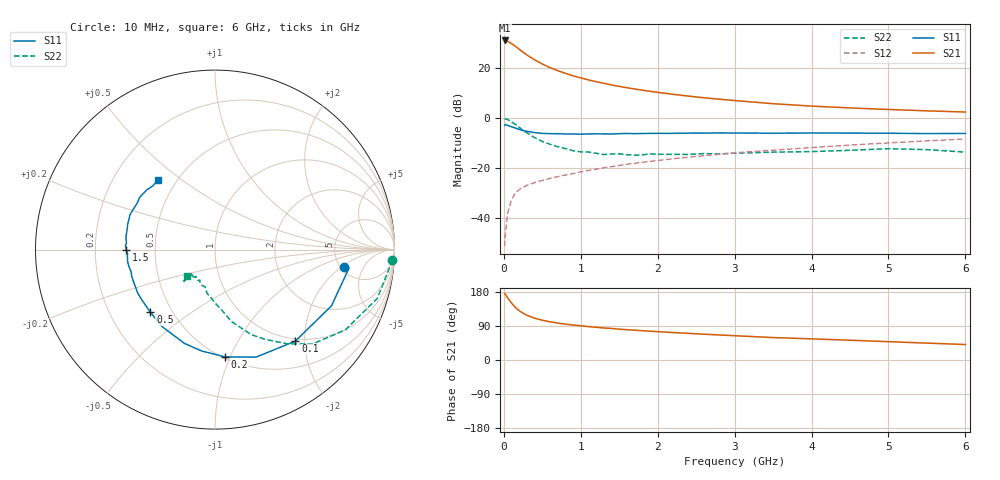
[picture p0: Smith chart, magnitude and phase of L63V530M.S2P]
!  INFINEON TECHNOLOGIES Small Signal Semiconductors
! BFR380L3 , Si-NPN RF-Transistor in TSLP-3-1
!  Vce=3.5 V,  Ic=30 mA
! Common Emitter S-Parameters:  07. March 2005
#  GHz  S  MA  R  50
! f  S11  S21  S12  S22
! GHz  Mag  Ang  Mag  Ang  Mag  Ang  Mag  Ang
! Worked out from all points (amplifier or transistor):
!   36 points, 10 MHz to 6 GHz, reference 50 ohm
!   highest |S21| = 31.1 dB at 10 MHz (marker M1)
!   |S21| within 3 dB of that: start of sweep to 178 MHz
!   unconditionally stable (mu >= 1): 1.886 GHz to 4.814 GHz
!   at 250 MHz: K = 0.40, MSG = 27.0 dB, |S12| = -27.6 dB
!   at 1.4 GHz: K = 0.96, MSG = 16.3 dB, |S12| = -19.3 dB
!   at 6 GHz: K = 0.98, MSG = 5.4 dB, |S12| = -8.2 dB
!   S11 on the Smith chart (normalised r, x): 10 MHz: 5.40, -2.20; 100 MHz: 0.96, -1.81; 200 MHz: 0.51, -0.96; 500 MHz: 0.38, -0.35; 1.5 GHz: 0.34, +0.00; 6 GHz: 0.40, +0.41
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0.01  0.7268 -7.6  35.98 174.8  0.0028 75.2  0.9905 -3.3
0.02  0.754 -7.8  35.84 173.5  0.005 88.7  0.9731 -6.8
0.05  0.7206 -25.8  34.55 163.9  0.0128 78.7  0.9446 -16.7
0.1  0.6786 -48.7  31.2 150.1  0.024 68.4  0.853 -31.6
0.15  0.6412 -69.1  27.54 138.7  0.0321 62.0  0.7556 -44.2
0.2  0.6005 -84.6  23.95 130.0  0.0378 58.2  0.6602 -52.6
0.25  0.5696 -97.5  20.99 123.5  0.0419 55.0  0.5729 -60.8
0.3  0.5497 -108.1  18.43 118.1  0.0459 54.0  0.515 -66.9
0.4  0.5204 -124.6  14.76 110.3  0.0522 52.9  0.4113 -77.1
0.5  0.5013 -135.9  12.2 105.0  0.0575 53.4  0.346 -82.8
0.6  0.4948 -144.9  10.32 100.7  0.0631 54.8  0.3041 -88.8
0.8  0.4883 -157.0  7.931 94.6  0.0738 57.2  0.2486 -99.9
0.9  0.4873 -162.3  7.075 92.3  0.0788 58.3  0.2258 -103.8
1.1  0.4887 -168.9  5.865 88.1  0.0912 60.2  0.2128 -109.6
1.5  0.4943 180.0  4.36 81.4  0.1147 62.7  0.1959 -119.9
1.9  0.5017 172.0  3.468 76.0  0.1382 63.8  0.1951 -128.2
2.2  0.5024 166.9  3.021 72.4  0.1562 64.0  0.191 -128.9
2.8  0.5121 157.7  2.413 66.1  0.1918 64.4  0.1949 -135.8
3.5  0.505 148.9  1.963 59.2  0.2315 62.7  0.2114 -135.1
4.5  0.5079 142.6  1.616 52.2  0.2921 61.5  0.2305 -135.0
5.5  0.4963 134.5  1.413 44.6  0.3549 58.1  0.2375 -134.6
6  0.5004 129.5  1.338 40.8  0.3869 56.0  0.2117 -136.4
